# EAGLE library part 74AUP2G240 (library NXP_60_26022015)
Low-power dual inverting buffer/line driver; 3-state The 74AUP2G240 provides the dual inverting buffer/line driver with 3-state output. The 3-state output is controlled by the output enable input (nOE). A HIGH level at pin nOE causes the output to assume a high-impedance OFF-state. Schmitt-trigger action at all inputs makes the circuit tolerant to slower input rise and fall times across the entire VCC range from 0.8 V to 3.6 V. This device ensures a very low static and dynamic power consumption across the entire VCC range from 0.8 V to 3.6 V. This device is fully specified for partial Power-down applications using IOFF. The IOFF circuitry disables the output, preventing the damaging backflow current through the device when it is powered down. This device has the input-disable feature, which allows floating input signals. The inputs are disabled when the output enable input nOE is HIGH.. AAL Eindhoven MK
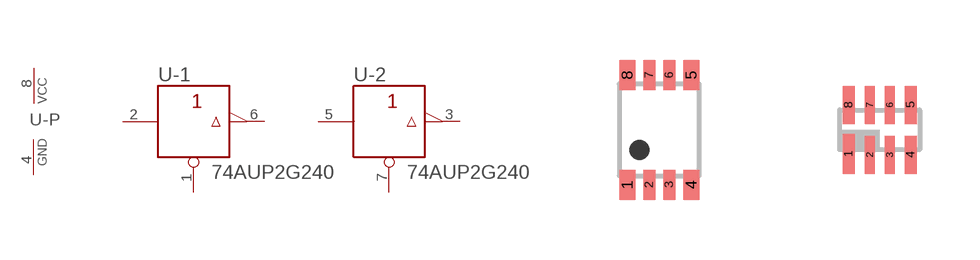
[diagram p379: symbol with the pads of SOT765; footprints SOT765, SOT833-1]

Designator prefix U; gates -P=PWRN -1=INVERTER_OE -2=INVERTER_OE

## 74AUP2G240DC  [SOT765]
1  -1:!OE  in
2  -1:A  in
3  -2:Y  out
4  -P:GND  pwr
5  -2:A  in
6  -1:Y  out
7  -2:!OE  in
8  -P:VCC  pwr

## 74AUP2G240GT  [SOT833-1]
Pads as for SOT765

## 74AUP2G240GF  [SOT1089-1]
Pads as for SOT765

## 74AUP2G240GD  [SOT996-2/3]
Pads as for SOT765

## 74AUP2G240GM  [SOT902-1/2/3]
Pads as for SOT765

## 74AUP2G240GS  [SOT1203]
Pads as for SOT765

## Footprint SOT765 (pad centres in mm)
SOT765 VSSOP8: plastic very thin shrink small outline package; 8 leads; body width 2.3 mm JEDEC: MO-187 IEC: -- JEITA: --
smd 0.4 x 0.75: 1 -0.8,-1.375; 4 0.8,-1.375; 5 0.8,1.375; 8 -0.8,1.375
smd 0.3 x 0.75: 2 -0.25,-1.375; 3 0.25,-1.375; 6 0.25,1.375; 7 -0.25,1.375

## Footprint SOT833-1 (pad centres in mm)
SOT833-1 XSON8: plastic extremely thin small outline package; no leads; 8 terminals; body 1 x 1.95 x 0.5 mm JEDEC: MO-252 IEC: -- JEITA: --
smd 0.3 x 1: 1 -0.775,-0.6
smd 0.25 x 0.95: 2 -0.25,-0.625; 3 0.25,-0.625; 6 0.25,0.625; 7 -0.25,0.625
smd 0.3 x 0.95: 4 0.775,-0.625; 5 0.775,0.625; 8 -0.775,0.625

## Footprint SOT1089-1 (pad centres in mm)
SOT1089-1 XSON8: plastic, extremely thin small outline package; no leads; 8 terminals; body 1 x 1.35 x 0.5 mm JEDEC: -- IEC: -- JEITA: --
smd 0.15 x 0.5: 1 -0.525,-0.35; 2 -0.175,-0.35; 3 0.175,-0.35; 4 0.525,-0.35; 5 0.525,0.35; 6 0.175,0.35; 7 -0.175,0.35; 8 -0.525,0.35

## Footprint SOT996-2/3 (pad centres in mm)
SOT996-2/3 XSON8U: plastic extremely thin small outline package; no leads;8 terminals; UTLP based; body 3 x 2 x 0.5 mm JEDEC: IEC: -- JEITA: --
smd 0.25 x 1.1: 1 -0.75,-1.45
smd 0.25 x 1: 2 -0.25,-1.5; 3 0.25,-1.5; 4 0.75,-1.5; 5 0.75,1.5; 6 0.25,1.5; 7 -0.25,1.5; 8 -0.75,1.5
